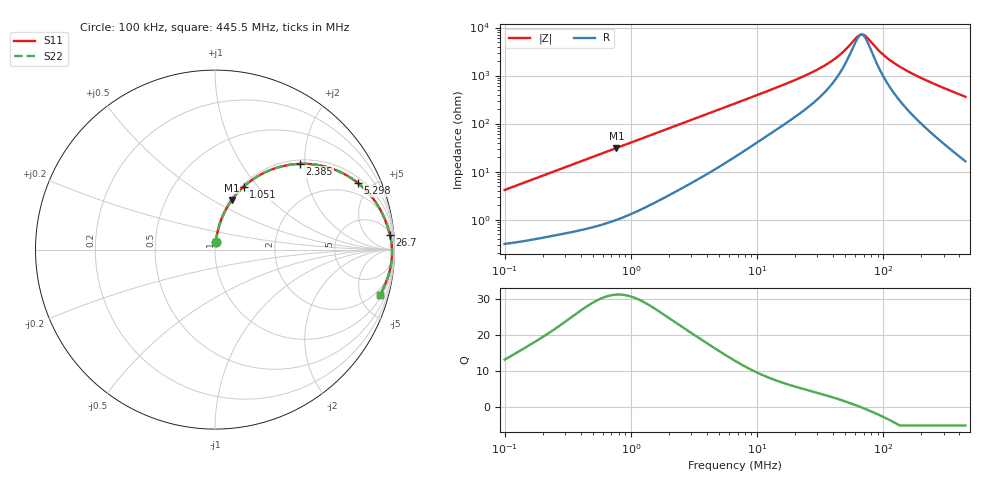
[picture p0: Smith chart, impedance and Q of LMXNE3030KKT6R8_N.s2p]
! LMXNE3030KKT6R8_N  S-PARAMETER MODEL  ( General Type )
! Model Generated by TAIYO YUDEN Corporation (https://www.yuden.co.jp/en/)
! Version 1.0
! TAIYO YUDEN Control No. 191023NI43SB-FBB
! Copyright(c) 2019 TAIYO YUDEN CO.,LTD. All Rights Reserved.
! Product Description (link to TY-COMPAS)
! https://ds.yuden.co.jp/TYCOMPAS/or/detail?pn=LMXNE3030KKT6R8MN&u=M
! Products Name : Inductors
! Characteristics :
!  Inductance : 6.8 uH , SRF(min) : 44 MHz , DC Resistance(max) : 0.3 Ohm
!  Rated Current : Saturation :700 mA , Temp Rise : 745 mA (40 degC)
!  Case Size : 3.0 x 3.0 / 0.118 x 0.118 [mm/inch] , Thickness : 1 / 0.039 [mm/inch]
!  (Conditions: Temperature = 25 degC , DC Bias Current/Voltage = 0A / 0V)
! External Node Assignments :
!  1  o---GGG---o  2
! GND o---------o GND
! Frequency Range : 0.1MHz  -  445.549718MHz  [ 402 STEP ]
# MHz S RI R 50
! Freq[MHz].  S11 Real  S11 Imag  S21 Real  S21 Imag  S12 Real  S12 Imag  S22 Real  S22 Imag
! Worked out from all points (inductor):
!   401 points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, 100 kHz to 445.5 MHz, reference 50 ohm
!   read as one part in series: L = 6.56 uH near 104.3 kHz
!   highest Q = 31.3 at 767.1 kHz (marker M1), where L = 6.4 uH
!   self-resonance near 66.99 MHz
!   S11 on the Smith chart (normalised r, x): 100 kHz: 1.01, +0.08; 1.051 MHz: 1.03, +0.84; 2.385 MHz: 1.08, +1.89; 5.298 MHz: 1.28, +4.16; 26.7 MHz: 6, +22; 445.5 MHz: 1.33, -7.22
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0.1  0.0048 0.041  0.9952 -0.041  0.9952 -0.041  0.0048 0.041
0.408498  0.0322 0.1591  0.9678 -0.1591  0.9678 -0.1591  0.0322 0.1591
0.767109  0.0943 0.2768  0.9057 -0.2768  0.9057 -0.2768  0.0943 0.2768
1.051213  0.1591 0.3498  0.8409 -0.3498  0.8409 -0.3498  0.1591 0.3498
1.668708  0.3139 0.4457  0.6861 -0.4457  0.6861 -0.4457  0.3139 0.4457
2.384835  0.4742 0.4781  0.5258 -0.4781  0.5258 -0.4781  0.4742 0.4781
3.408289  0.6381 0.4555  0.3619 -0.4555  0.3619 -0.4555  0.6381 0.4555
5.297896  0.7976 0.37  0.2024 -0.37  0.2024 -0.37  0.7976 0.37
6.81664  0.8592 0.3108  0.1408 -0.3108  0.1408 -0.3108  0.8592 0.3108
12.01907  0.9364 0.1919  0.0636 -0.1919  0.0636 -0.1919  0.9364 0.1919
26.70029  0.9746 0.0818  0.0254 -0.0818  0.0254 -0.0818  0.9746 0.0818
27.26705  0.9751 0.0796  0.0249 -0.0796  0.0249 -0.0796  0.9751 0.0796
42.38432  0.983 0.038  0.017 -0.038  0.017 -0.038  0.983 0.038
50.13987  0.9846 0.0238  0.0154 -0.0238  0.0154 -0.0238  0.9846 0.0238
61.85938  0.9859 0.00651  0.0141 -0.00651  0.0141 -0.00651  0.9859 0.00651
65.88284  0.9862 0.00137  0.0138 -0.00137  0.0138 -0.00137  0.9862 0.00137
73.1785  0.9864 -0.00724  0.0136 0.00724  0.0136 0.00724  0.9864 -0.00724
92.19941  0.9862 -0.0267  0.0138 0.0267  0.0138 0.0267  0.9862 -0.0267
111.3854  0.9853 -0.0437  0.0147 0.0437  0.0147 0.0437  0.9853 -0.0437
140.3372  0.9829 -0.0665  0.0171 0.0665  0.0171 0.0665  0.9829 -0.0665
192.3121  0.9766 -0.1033  0.0234 0.1033  0.0234 0.1033  0.9766 -0.1033
445.5497  0.9192 -0.2508  0.0808 0.2508  0.0808 0.2508  0.9192 -0.2508
